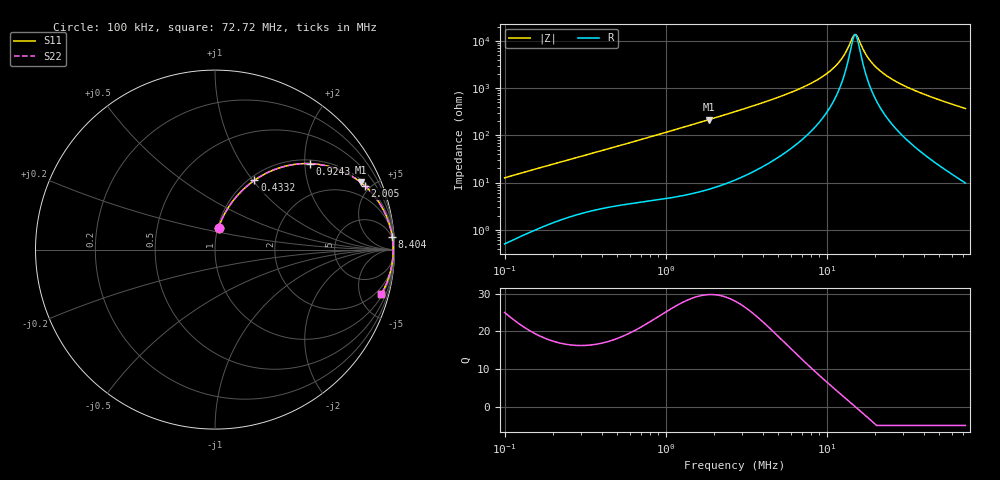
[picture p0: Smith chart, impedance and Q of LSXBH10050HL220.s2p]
! LSXBH10050HL220  S-PARAMETER MODEL  ( General Type )
! Model Generated by TAIYO YUDEN Corporation (http://www.ty-top.com)
! Version 3.0
! TAIYO YUDEN Control No. 180118NI43SB-FBB
! Copyright(c) 2007 TAIYO YUDEN CO.,LTD. All Rights Reserved.
! Product Description (link to TY-COMPAS)
! https://ds.yuden.co.jp/TYCOMPAS/or/detail?pn=LSXBH10050HL220M&u=M
! Products Name : Inductors
! Characteristics :
!  Inductance : 22 uH , SRF(min) : 10 MHz , DC Resistance(max) : 0.0585 Ohm
!  Rated Current : Saturation :2600 mA , Temp Rise : 2500 mA (40 degC)
!  Case Size : 10.0 x 9.8 / 0.394 x 0.386 [mm/inch] , Thickness : 5 / 0.197 [mm/inch]
!  (Conditions: Temperature = 25 degC , DC Bias Current/Voltage = 0A / 0V)
! External Node Assignments :
!  1  o---GGG---o  2
! GND o---------o GND
! Frequency Range : 0.1MHz  -  72.722828MHz  [ 402 STEP ]
# MHz S RI R 50
! Freq[MHz].  S11 Real  S11 Imag  S21 Real  S21 Imag  S12 Real  S12 Imag  S22 Real  S22 Imag
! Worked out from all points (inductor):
!   401 points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, 100 kHz to 72.72 MHz, reference 50 ohm
!   read as one part in series: L = 19.9 uH near 103.3 kHz
!   highest Q = 29.8 at 1.846 MHz (marker M1), where L = 18.4 uH
!   self-resonance near 14.96 MHz
!   S11 on the Smith chart (normalised r, x): 100 kHz: 1.01, +0.25; 433.2 kHz: 1.06, +1.02; 924.3 kHz: 1.09, +2.13; 2.005 MHz: 1.16, +4.64; 8.404 MHz: 4, +27; 72.72 MHz: 1.20, -7.37
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0.1  0.0203 0.1226  0.9797 -0.1226  0.9797 -0.1226  0.0203 0.1226
0.30153  0.1303 0.3073  0.8697 -0.3073  0.8697 -0.3073  0.1303 0.3073
0.433233  0.2196 0.386  0.7804 -0.386  0.7804 -0.386  0.2196 0.386
0.909201  0.5218 0.4792  0.4782 -0.4792  0.4782 -0.4792  0.5218 0.4792
0.924302  0.5297 0.4789  0.4703 -0.4789  0.4703 -0.4789  0.5297 0.4789
1.846245  0.8117 0.3745  0.1883 -0.3745  0.1883 -0.3745  0.8117 0.3745
2.00475  0.8353 0.3545  0.1647 -0.3545  0.1647 -0.3545  0.8353 0.3545
2.741508  0.9039 0.2774  0.0961 -0.2774  0.0961 -0.2774  0.9039 0.2774
5.211977  0.9707 0.1431  0.0293 -0.1431  0.0293 -0.1431  0.9707 0.1431
8.131398  0.9867 0.0751  0.0133 -0.0751  0.0133 -0.0751  0.9867 0.0751
8.403759  0.9874 0.0707  0.0126 -0.0707  0.0126 -0.0707  0.9874 0.0707
10.07325  0.9903 0.0474  0.00969 -0.0474  0.00969 -0.0474  0.9903 0.0474
11.68307  0.9918 0.0294  0.00822 -0.0294  0.00822 -0.0294  0.9918 0.0294
12.89681  0.9924 0.0178  0.00763 -0.0178  0.00763 -0.0178  0.9924 0.0178
14.4731  0.9927 0.00444  0.00729 -0.00444  0.00729 -0.00444  0.9927 0.00444
14.95787  0.9927 0.000637  0.00726 -0.000637  0.00726 -0.000637  0.9927 0.000637
15.45888  0.9927 -0.00317  0.00727 0.00317  0.00727 0.00317  0.9927 -0.00317
17.34832  0.9925 -0.0165  0.00751 0.0165  0.00751 0.0165  0.9925 -0.0165
18.83772  0.9921 -0.0262  0.00791 0.0262  0.00791 0.0262  0.9921 -0.0262
24.51857  0.9894 -0.0585  0.0106 0.0585  0.0106 0.0585  0.9894 -0.0585
37.62735  0.9782 -0.1196  0.0218 0.1196  0.0218 0.1196  0.9782 -0.1196
72.72283  0.9258 -0.2492  0.0742 0.2492  0.0742 0.2492  0.9258 -0.2492
